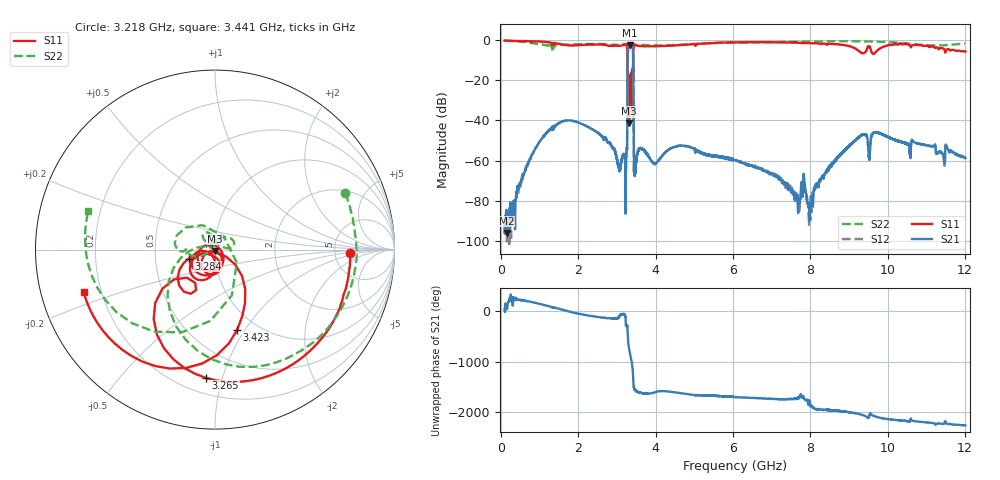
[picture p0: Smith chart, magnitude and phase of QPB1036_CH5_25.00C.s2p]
! TDS: K:\Engsetup\Winsaw\QPB1036_ALL
! Channel 1
! Ports=1 2
! seg 1=100.000000 1100.000000 101
! seg 2=1101.000000 1501.000000 401
! seg 3=1502.000000 2502.000000 101
! seg 4=2503.000000 3803.000000 1301
! seg 5=3804.000000 5004.000000 121
! seg 6=5005.000000 6005.000000 1001
! seg 7=6006.000000 8406.000000 241
! seg 8=8407.000000 10607.000000 2201
! seg 9=10608.000000 12008.000000 141
! Points=5609
! FailCode=0
! Topology=ALL_SE(12)
!VNA Cal loaded =QPB1036_ALL_25C
!PS1(V)= 5.000
!PS(mA)= 0.500
!PS2(V)= 1.170
!PS(mA)= -0.100
!PS3(V)= 0.630
!PS(mA)= 0.100
!PS4(V)= 1.170
!PS(mA)= -0.100
!Temp (C)= 25.00
# MHz S DB R 50
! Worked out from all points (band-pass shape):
!   5609 points, 100 MHz to 12.01 GHz, reference 50 ohm
!   highest |S21| = -2.54 dB at 3.337 GHz (marker M1); lowest = -95.7 dB at 160 MHz (marker M2)
!   |S21| within 3 dB of the highest: 3.287 GHz to 3.418 GHz (131.3 MHz wide, 3.92 % of centre)
!   lowest |S11| = -41.4 dB at 3.318 GHz (marker M3), VSWR 1.02, Z = 49.8 - j0.828 ohm
!   |S11| at or under -10 dB: 3.274 GHz to 3.421 GHz (147.1 MHz wide, 4.39 % of centre)
!   |S22| runs from -34.3 to -0.3 dB; largest |S21 - S12| = 0.0061
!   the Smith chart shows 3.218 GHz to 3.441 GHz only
!   S11 on the Smith chart (normalised r, x): 3.218 GHz: 7.07, -0.58; 3.265 GHz: 0.30, -0.88; 3.284 GHz: 0.74, -0.08; 3.423 GHz: 0.81, -0.92; 3.441 GHz: 0.13, -0.15
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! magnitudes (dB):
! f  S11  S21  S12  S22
! 100 MHz  -0.4  -95.7  -91.8  -0.3
! 160 MHz  -0.5  -95.7  -100.1  -0.4
! 1.235 GHz  -1.2  -45.3  -45.3  -2.8
! 2.092 GHz  -2.5  -41.7  -41.7  -2.1
! 3.218 GHz  -2.5  -62.7  -63.0  -2.0
! 3.243 GHz  -2.3  -58.7  -58.6  -2.1
! 3.265 GHz  -2.9  -54.4  -54.4  -2.6
! 3.284 GHz  -16.1  -6.6  -6.5  -23.1
! 3.318 GHz  -41.4  -2.8  -2.8  -23.9
! 3.337 GHz  -18.4  -2.5  -2.5  -28.1
! 3.398 GHz  -29.1  -3.2  -3.2  -29.6
! 3.423 GHz  -6.7  -9.7  -9.7  -21.0
! 3.441 GHz  -2.3  -65.0  -65.5  -2.6
! 3.467 GHz  -2.5  -66.1  -67.4  -2.5
! 3.598 GHz  -3.1  -53.8  -54.0  -2.5
! 4.074 GHz  -3.1  -60.1  -59.5  -2.7
! 6.056 GHz  -1.2  -59.6  -59.8  -1.4
! 8.046 GHz  -1.7  -82.2  -79.1  -0.8
! 9.302 GHz  -6.3  -47.6  -47.5  -0.7
! 9.521 GHz  -3.6  -59.0  -58.9  -0.8
! 10.02 GHz  -2.4  -48.3  -48.3  -1.2
! 12.01 GHz  -5.8  -58.7  -58.8  -1.8
